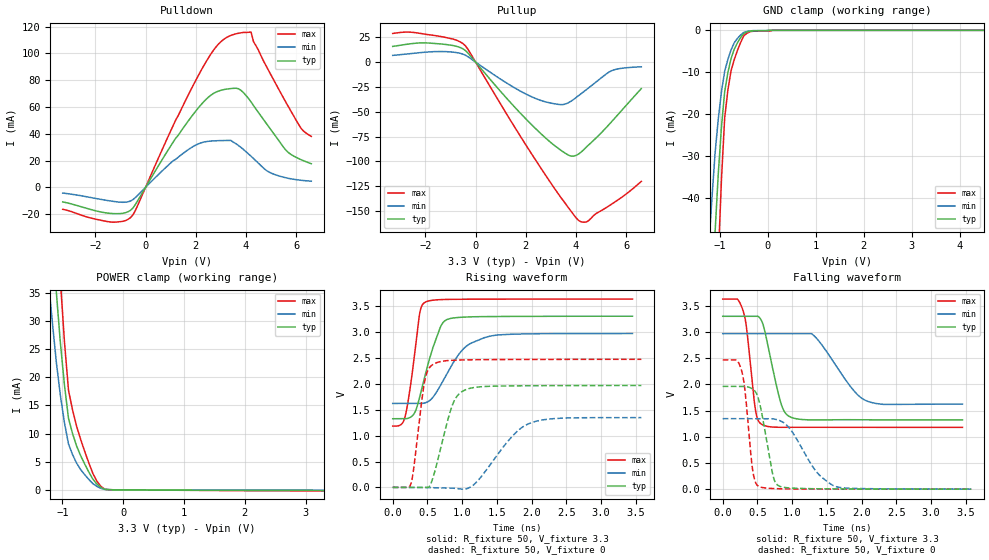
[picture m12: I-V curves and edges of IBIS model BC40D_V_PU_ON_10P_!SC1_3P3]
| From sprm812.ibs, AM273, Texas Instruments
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|   Model Cell BC40D_V_PU_ON_10P_!SC1_3P3
|BC40D_V_PU_ON_10P_!SC1_3P3
[Model]   BC40D_V_PU_ON_10P_!SC1_3P3
Model_type   I/O
Polarity   Non-Inverting
Enable   Active-Low
Vinl =  0.8V
Vinh =  2V
Cref =  15pF
Rref =  100.0000M
Vref =  0V
Vmeas =  1.65
C_comp   2.059994p   1.912853p   2.135747p
|[Input load] weak_pu_on
|[Output drive] fast
|[supplytol] 10
|[temp] ind
[Model Spec]
Vinl   0.8V   0.8V   0.8V
Vinh   2V   2V   2V
[Temperature Range]   25   125   -40
[Voltage Range]   3.3   2.97   3.63
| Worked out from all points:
|   slope of the pulldown table from 0 to 0.495 V, typ, clamps not added: 31.8 ohm
|   slope of the pullup table from 0 to 0.495 V, typ, clamps not added: 33.3 ohm
|   GND clamp passes 1 mA (typ) near -0.52 V on its own axis
|   POWER clamp passes 1 mA (typ) near -0.43 V on its own axis
|   rising waveform, R_fixture 50, V_fixture 3.3: 20-80 % time 251ps typ, 384ps min, 142ps max; typ from 1.32 V to 3.3 V
|   rising waveform, R_fixture 50, V_fixture 0: 20-80 % time 232ps typ, 477ps min, 136ps max; typ from 0.002 V to 1.97 V
|   falling waveform, R_fixture 50, V_fixture 3.3: 20-80 % time 196ps typ, 423ps min, 118ps max; typ from 3.3 V to 1.32 V
|   falling waveform, R_fixture 50, V_fixture 0: 20-80 % time 159ps typ, 382ps min, 106ps max; typ from 1.96 V to 0.002 V
| Nom Voltages:
|   VDD=1.1001, VDDS=3.3, VDDS18=1.8, ESD_BIASFET=0, VSS=0, VSSS=0
| Min Voltages:
|   VDD=0.99, VDDS=2.97, VDDS18=1.62, ESD_BIASFET=0, VSS=0, VSSS=0
| Max Voltages:
|   VDD=1.21, VDDS=3.63, VDDS18=1.98, ESD_BIASFET=0, VSS=0, VSSS=0
[POWER_clamp]
|   voltage   I(typ)   I(min)   I(max)
-3.3V     446.9mA    419.5mA    603.9mA
-1.233V   56.55mA    37.52mA    80.26mA
-1.167V   45.63mA    29.9mA     65.05mA
-1.1V     35.1mA     22.66mA    50.24mA
-1.033V   26.08mA    16.76mA    37.18mA
-966.7mV  18.62mA    11.92mA    26.33mA
-900mV    12.7mA     8.149mA    17.69mA
-833.3mV  10mA       6.265mA    14.21mA
-766.7mV  7.795mA    4.753mA    11.3mA
-566.7mV  3.199mA    1.871mA    4.823mA
-366.7mV  433.5uA    268.4uA    618.3uA
3.3V      -100.3uA   -83.23uA   -188.3uA
[Pulldown]
|   voltage   I(typ)   I(min)   I(max)
-3.3V     -10.92mA   -4.307mA   -16.45mA
-1.4V     -19.52mA   -10.22mA   -25.94mA
-600mV    -17.22mA   -10.25mA   -22.66mA
1.1V      33.8mA     19.88mA    46.22mA
2.1V      59.3mA     32.44mA    83.48mA
2.9V      71.86mA    34.84mA    107mA
3.5V      73.95mA    33.66mA    114.2mA
4.2V      63.8mA     23.19mA    116mA
4.9V      45.33mA    11.53mA    87.2mA
5.6V      27.47mA    7.046mA    63.1mA
6.2V      20.56mA    5.221mA    43.87mA
6.6V      17.6mA     4.555mA    38.05mA
[Pullup]
|   voltage   I(typ)   I(min)   I(max)
-3.3V     15.77mA    6.741mA    28.8mA
-1.9V     19.23mA    10.15mA    27.67mA
-900mV    16.69mA    10.02mA    23.17mA
-400mV    11.53mA    6.853mA    16.25mA
1.3V      -38.16mA   -22.04mA   -54.88mA
2.3V      -64.7mA    -35.66mA   -95.04mA
3.4V      -88.76mA   -42.82mA   -136.4mA
3.8V      -94.64mA   -39.36mA   -150mA
4.1V      -92.53mA   -33.79mA   -159.3mA
4.4V      -85.77mA   -27.94mA   -161mA
5.4V      -60.46mA   -8.849mA   -143.2mA
6.6V      -26.71mA   -4.741mA   -120mA
[GND_clamp]
|   voltage   I(typ)   I(min)   I(max)
-3.3V     -787.2mA   -607.8mA   -1.235A
-1.233V   -85.67mA   -52.14mA   -138.8mA
-1.167V   -66.48mA   -40.37mA   -107.8mA
-1.1V     -48.26mA   -29.37mA   -78.02mA
-1.033V   -34.3mA    -21.2mA    -54.63mA
-966.7mV  -23.1mA    -14.67mA   -35.61mA
-900mV    -14.66mA   -9.802mA   -20.96mA
-833.3mV  -10.12mA   -6.954mA   -14.3mA
-700mV    -4.501mA   -2.964mA   -6.982mA
-500mV    -717.7uA   -486.4uA   -1.28mA
100mV     0A         0A         0A
6.6V      0A         0A         0A
[Ramp]
| variable   typ   min   max
dV/dt_f  1.1950496/0.19764937n 0.83550004/0.43952187n  1.4746494/0.11842933n
dV/dt_r  1.1911253/0.23433637n 0.82860168/0.48872151n  1.4896931/0.13693182n
R_load = 50
[Rising Waveform]
R_fixture = 50
V_fixture = 3.3
V_fixture_min = 2.97
V_fixture_max = 3.63
|   time   V(typ)   V(min)   V(max)
0s        1.324V     1.618V     1.183V
179.3ps   1.324V     1.618V     1.369V
305.5ps   1.417V     1.618V     2.459V
385.5ps   1.726V     1.618V     3.332V
470.7ps   2.181V     1.632V     3.571V
684ps     3.082V     1.957V     3.619V
810.8ps   3.249V     2.263V     3.624V
1.057ns   3.284V     2.718V     3.627V
1.408ns   3.293V     2.917V     3.628V
3.453ns   3.299V     2.966V     3.63V
[Rising Waveform]
R_fixture = 50
V_fixture = 0
V_fixture_min = 0
V_fixture_max = 0
|   time   V(typ)   V(min)   V(max)
0s        2.484mV    0V         3.666mV
261.9ps   2.484mV    0V         69.24mV
302ps     2.484mV    0V         363.3mV
458.8ps   2.484mV    0V         2.037V
523.9ps   12.11mV    -2.334mV   2.298V
595.8ps   259.4mV    -4.175mV   2.383V
855.5ps   1.573V     -12.76mV   2.45V
1.044ns   1.879V     -29.25mV   2.458V
1.976ns   1.96V      1.238V     2.467V
3.581ns   1.965V     1.345V     2.469V
[Falling Waveform]
R_fixture = 50
V_fixture = 3.3
V_fixture_min = 2.97
V_fixture_max = 3.63
|   time   V(typ)   V(min)   V(max)
0s        3.301V     2.97V      3.629V
295.6ps   3.301V     2.97V      3.399V
346.7ps   3.301V     2.97V      3.046V
472.1ps   3.301V     2.97V      1.511V
569.4ps   3.187V     2.97V      1.233V
833.3ps   1.664V     2.97V      1.183V
967.6ps   1.384V     2.97V      1.183V
1.307ns   1.323V     2.939V     1.183V
2.078ns   1.326V     1.683V     1.182V
3.453ns   1.324V     1.626V     1.182V
[Falling Waveform]
R_fixture = 50
V_fixture = 0
V_fixture_min = 0
V_fixture_max = 0
|   time   V(typ)   V(min)   V(max)
0s        1.964V     1.348V     2.469V
271.3ps   1.963V     1.348V     2.266V
323.1ps   1.962V     1.348V     1.859V
431.4ps   1.912V     1.348V     367.4mV
519.4ps   1.706V     1.348V     55.26mV
722.8ps   270.6mV    1.344V     14.62mV
816.2ps   59.94mV    1.313V     10.06mV
1.352ns   9.833mV    330.5mV    3.912mV
1.619ns   7.259mV    56.89mV    3.351mV
3.581ns   2.485mV    4.344mV    3.075mV
